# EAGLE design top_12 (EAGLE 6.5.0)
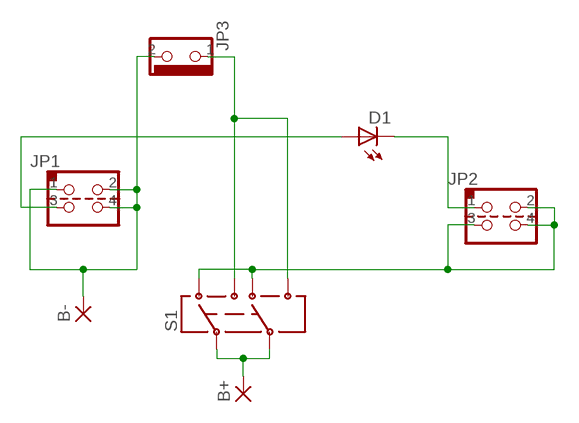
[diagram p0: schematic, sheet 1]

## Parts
B+  1,6/0,8  [1,6/0,8]
B-  1,6/0,8  [1,6/0,8]
D1  LED-1206  [LED-SMD-1206]
JP1  PINH_2X2-2MM  [2X2/2,0]
JP2  PINH_2X2-2MM  [2X2/2,0]
JP3  PINH_1X2-90°  [1X2/90]
S1  CL-SB-22B  [CL-SB-22B]

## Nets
N$1: B+.1(P) S1.2 S1.5
N$2: B-.1(P) JP1.1 JP1.2 JP1.4 JP3.2
N$3: JP2.2 JP2.3 JP2.4 S1.1 S1.4
N$4: JP3.1 S1.3 S1.6
N$5: D1.A JP1.3
N$7: D1.K(C) JP2.1

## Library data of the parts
B+ B- = wirepad:1,6/0,8: THROUGH-HOLE PAD
D1 = _dpa222:LED
JP1 JP2 = _dpa222:PINH_2X2
JP3 = _dpa222:PINH_1X2
S1 = _dpa222:CL-SB-22B

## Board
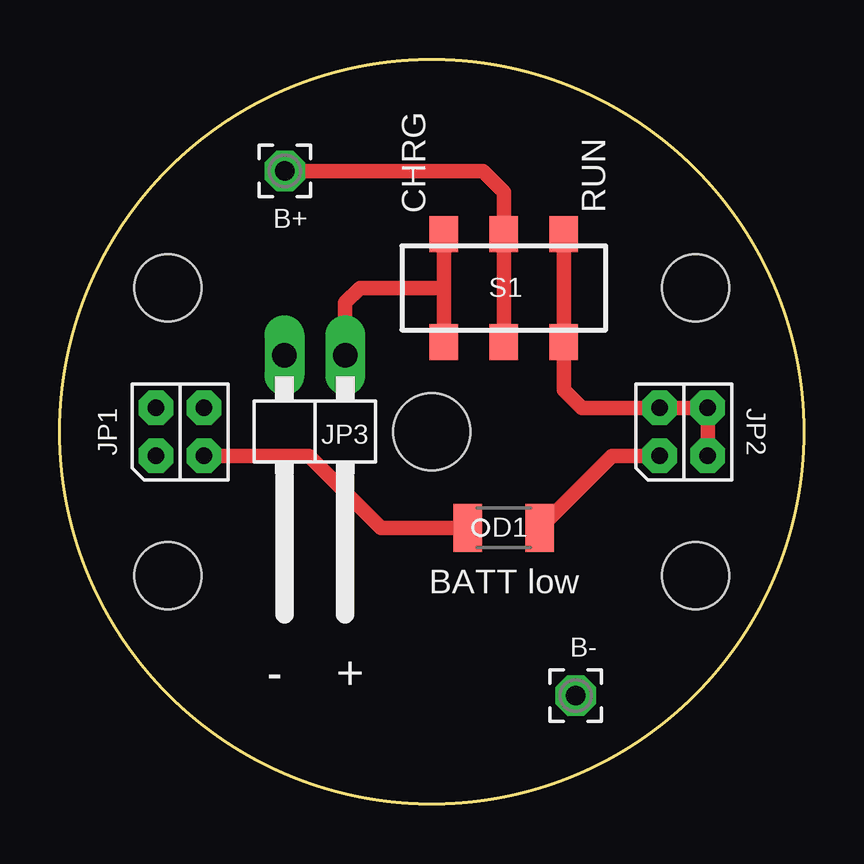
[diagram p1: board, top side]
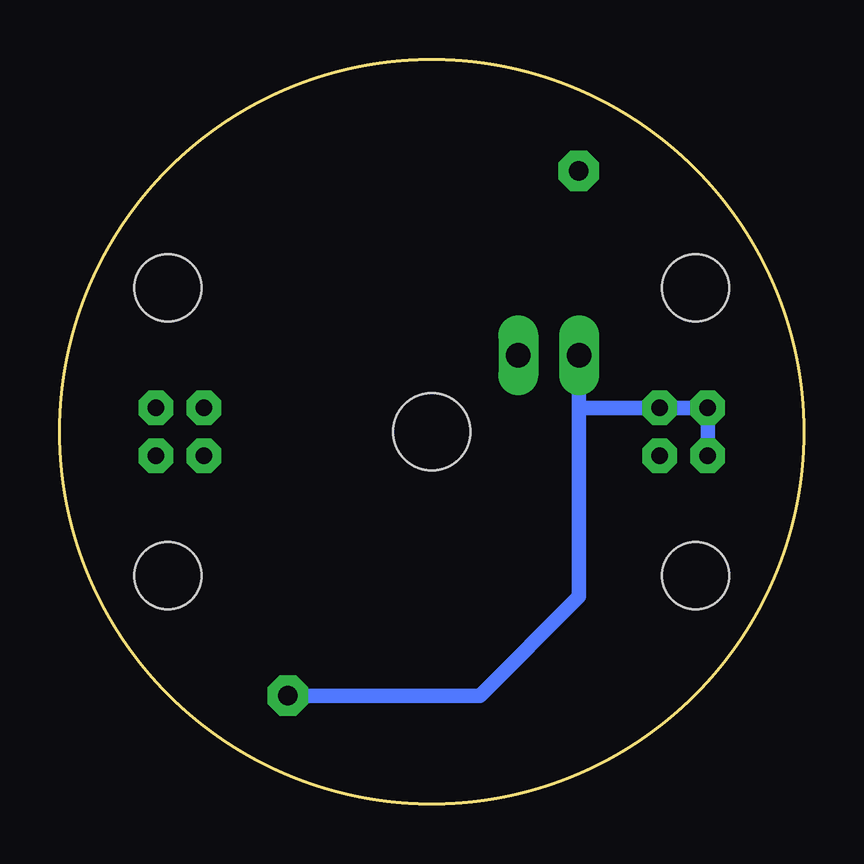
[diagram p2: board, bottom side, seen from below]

Size 31 x 31 mm. Coordinates in mm from the lower left corner, seen from the top.
Outline: circle at 15.5,15.5 radius 15.5
Copper layers (1*16): Top 0.035mm / dielectric 1.5mm / Bottom 0.035mm
Design rules "default *": minimum track width 10mil, minimum drill 24mil, track to track 8mil, track to pad 8mil, pad to pad 8mil, via to via 8mil, smd to smd 8mil, copper to edge 40mil, drill to drill 8mil, minimum pad ring 10mil, minimum via ring 8mil, stop-mask expansion 4mil, vias tented up to drill 0mil, thermal gap 10mil
Holes 3.2 mm at 15.5,15.5
Holes 2.8 mm at 4.5,21.5 26.5,9.5 26.5,21.5 4.5,9.5

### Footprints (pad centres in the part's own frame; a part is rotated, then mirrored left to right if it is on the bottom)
1,6/0,8 = drill 0.813 pad 1.676 octagon: 1 0,0
LED-SMD-1206 = smd 1.2 x 2: A -1.5,0; K 1.5,0
2X2/2,0 = drill 0.7 pad 1.422 octagon: 1 -1,-1; 2 -1,1; 3 1,-1; 4 1,1
1X2/90 = drill 1.016 pad 1.676 long: 1 -1.27,-3.81; 2 1.27,-3.81
CL-SB-22B = smd 1.2 x 1.5: 1 -2.5,2.25; 2 0,2.25; 3 2.5,2.25; 4 -2.5,-2.25; 5 0,-2.25; 6 2.5,-2.25

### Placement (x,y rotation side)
B+  9.38,26.38 0 top
B-  21.5,4.5 0 top
D1  18.5,11.5 0 top
JP1  5,15.5 0 top
JP2  26,15.5 0 top
JP3  10.62,14.88 180 top
S1  18.5,21.5 180 top

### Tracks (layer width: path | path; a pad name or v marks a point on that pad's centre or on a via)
N$1
  Top 0.61: S1.2 S1.5 18.5,25.5 17.62,26.38 B+.1
N$2
  Bottom 0.61: JP1.1 JP1.2 JP1.4 9.36,16.5 | JP3.2 9.36,16.5 | 9.36,16.5 9.36,8.64 13.5,4.5 B-.1
N$3
  Top 0.61: JP2.3 JP2.4 JP2.2 21.75,16.5 21,17.25 S1.1 S1.4
N$4
  Top 0.61: S1.3 16,21.5 | 16,21.5 S1.6 | JP3.1 11.89,20.89 12.5,21.5 16,21.5
N$5
  Top 0.61: JP1.3 10.38,14.5 13.38,11.5 D1.A
N$7
  Top 0.61: D1.K 23,14.5 JP2.1

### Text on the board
tNames: CHRG | RUN | BATT low | - | +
